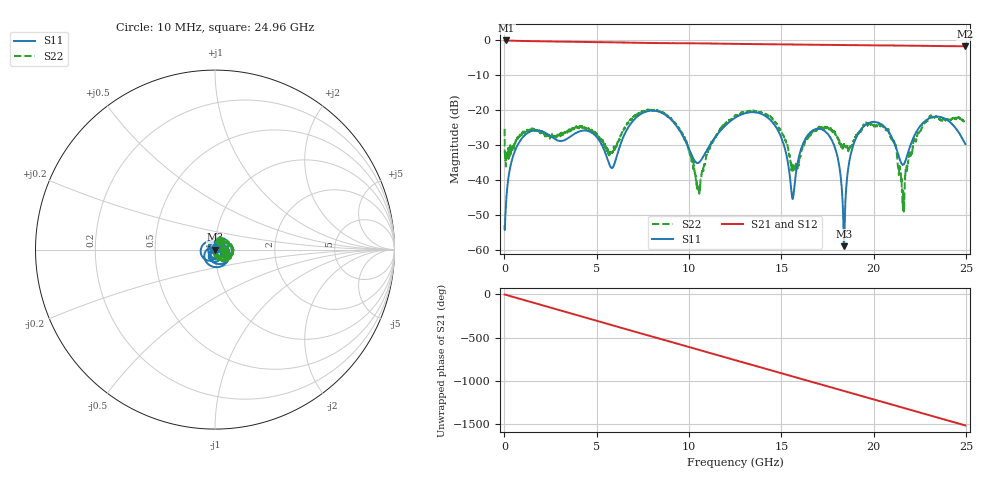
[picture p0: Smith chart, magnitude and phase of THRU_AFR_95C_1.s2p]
!Keysight Technologies,M9372A,MY54321388,A.12.55.09
!Automatic Fixture Removal (AFR)
!Date: Wednesday, May 22, 2019 8:34:25 AM
!S2P File: Measurements: S11,S21,S12,S22:
# MHz S  RI  R 50
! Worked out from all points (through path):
!   2496 points, 10 MHz to 24.96 GHz, reference 50 ohm
!   highest |S21| = -0.03 dB at 110 MHz (marker M1); lowest = -1.7 dB at 24.94 GHz (marker M2)
!   group delay of S21, straight-line fit = 169 ps
!   lowest |S11| = -58.8 dB at 18.39 GHz (marker M3), VSWR 1.00, Z = 50 - j0.108 ohm
!   |S11| at or under -10 dB: start of sweep to end of sweep
!   |S22| runs from -49.2 to -19.7 dB; largest |S21 - S12| = 1.4e-15
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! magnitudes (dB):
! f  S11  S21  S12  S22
! 10 MHz  -53.1  -0.1  -0.1  -25.3
! 110 MHz  -44.6  0.0  0.0  -33.9
! 430 MHz  -33.7  -0.1  -0.1  -30.5
! 1.1 GHz  -27.1  -0.2  -0.2  -26.2
! 4.17 GHz  -25.8  -0.4  -0.4  -24.5
! 5.83 GHz  -36.4  -0.6  -0.6  -32.1
! 6.94 GHz  -23.1  -0.7  -0.7  -22.1
! 8.33 GHz  -20.3  -0.8  -0.8  -20.1
! 9.75 GHz  -28.2  -0.8  -0.8  -28.3
! 10.49 GHz  -35.0  -0.9  -0.9  -42.2
! 12.49 GHz  -22.1  -1.0  -1.0  -21.5
! 14.57 GHz  -23.7  -1.1  -1.1  -22.7
! 15.61 GHz  -45.2  -1.2  -1.2  -37.2
! 16.65 GHz  -25.9  -1.2  -1.2  -26.4
! 17.82 GHz  -29.6  -1.3  -1.3  -26.0
! 18.39 GHz  -58.8  -1.3  -1.3  -29.6
! 19.16 GHz  -26.6  -1.4  -1.4  -26.6
! 20.81 GHz  -26.2  -1.5  -1.5  -25.7
! 21.59 GHz  -35.5  -1.5  -1.5  -42.5
! 22.99 GHz  -22.3  -1.6  -1.6  -22.0
! 24.94 GHz  -29.4  -1.7  -1.7  -23.1
! 24.96 GHz  -29.6  -1.7  -1.7  -23.0
